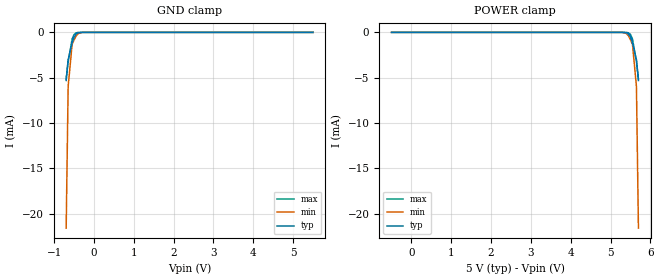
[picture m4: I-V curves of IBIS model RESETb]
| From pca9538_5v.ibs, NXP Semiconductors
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[Model]   RESETb
Model_type Input
Vinh=3.5
Vinl=1.5
C_comp   1.73p   1.7p   1.78p
[Temperature Range] 27   85   -40
[Voltage Range]   5   4.5   5.5
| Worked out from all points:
|   GND clamp passes 1 mA (typ) near -0.54 V on its own axis
[GND Clamp]
-700mV    -5.302mA   -21.58mA   -5.122mA
-650mV    -2.995mA   -5.963mA   -3.206mA
-550mV    -1.169mA   -1.297mA   -720.1uA
-500mV    -525.2uA   -816.9uA   -228.9uA
-450mV    -185.2uA   -388.2uA   -49.68uA
-400mV    -48.21uA   -135uA     -7.763uA
-250mV    -208.1nA   -1.277uA   -8.827nA
5.5V      106.9pA    399pA      72.28pA
[POWER Clamp]
-500mV    106.9pA    399pA      72.28pA
5.25V     -208nA     -1.277uA   -8.827nA
5.4V      -48.21uA   -135uA     -7.763uA
5.45V     -185.2uA   -388.2uA   -49.68uA
5.5V      -525.2uA   -816.9uA   -228.9uA
5.55V     -1.169mA   -1.297mA   -720.1uA
5.65V     -2.995mA   -5.963mA   -3.206mA
5.7V      -5.302mA   -21.58mA   -5.122mA
